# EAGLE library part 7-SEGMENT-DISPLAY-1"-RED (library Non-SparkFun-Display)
7-Segment Display 1" Red (COM-08546) EZ is for kits. Pads are only exposed on the bottom side to help prevent soldering in upside down.
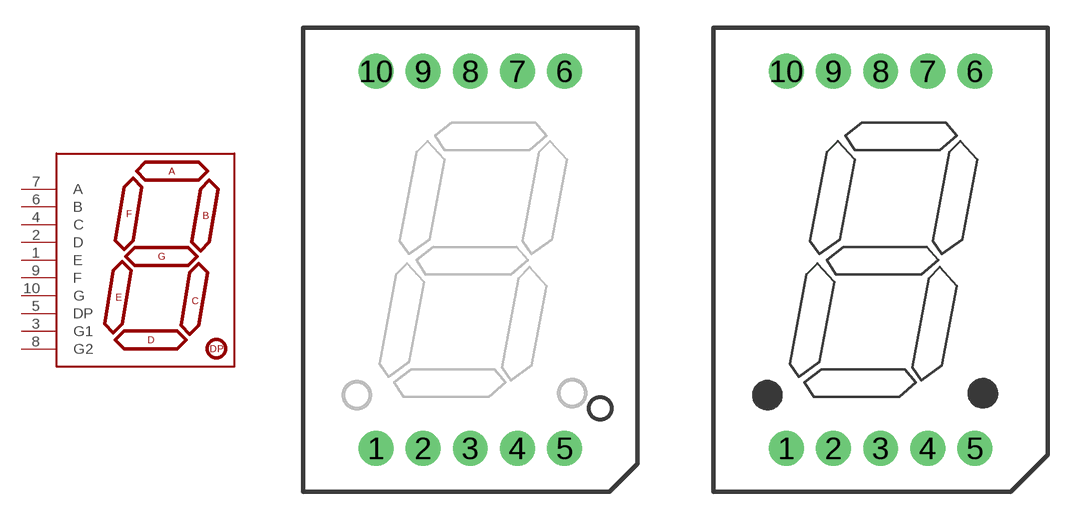
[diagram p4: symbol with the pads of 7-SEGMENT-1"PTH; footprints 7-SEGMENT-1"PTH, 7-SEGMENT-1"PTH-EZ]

Designator prefix -

## 7-SEGMENT-DISPLAY-1"-RED  [7-SEGMENT-1"PTH]
1  E
2  D
3  G1
4  C
5  DP
6  B
7  A
8  G2
9  F
10  G

## 7-SEGMENT-DISPLAY-1"-REDEZ  [7-SEGMENT-1"PTH-EZ]
Pads as for 7-SEGMENT-1"PTH

## Footprint 7-SEGMENT-1"PTH (pad centres in mm)
7 Segment display Storefront SKU#: COM-08546
drill 1 pad 1.88: 1 -5.08,-10.16; 2 -2.54,-10.16; 3 0,-10.16; 4 2.54,-10.16; 5 5.08,-10.16; 6 5.08,10.16; 7 2.54,10.16; 8 0,10.16; 9 -2.54,10.16; 10 -5.08,10.16

## Footprint 7-SEGMENT-1"PTH-EZ (pad centres in mm)
drill 1 pad 1.88: 1 -5.08,-10.16; 2 -2.54,-10.16; 3 0,-10.16; 4 2.54,-10.16; 5 5.08,-10.16; 6 5.08,10.16; 7 2.54,10.16; 8 0,10.16; 9 -2.54,10.16; 10 -5.08,10.16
